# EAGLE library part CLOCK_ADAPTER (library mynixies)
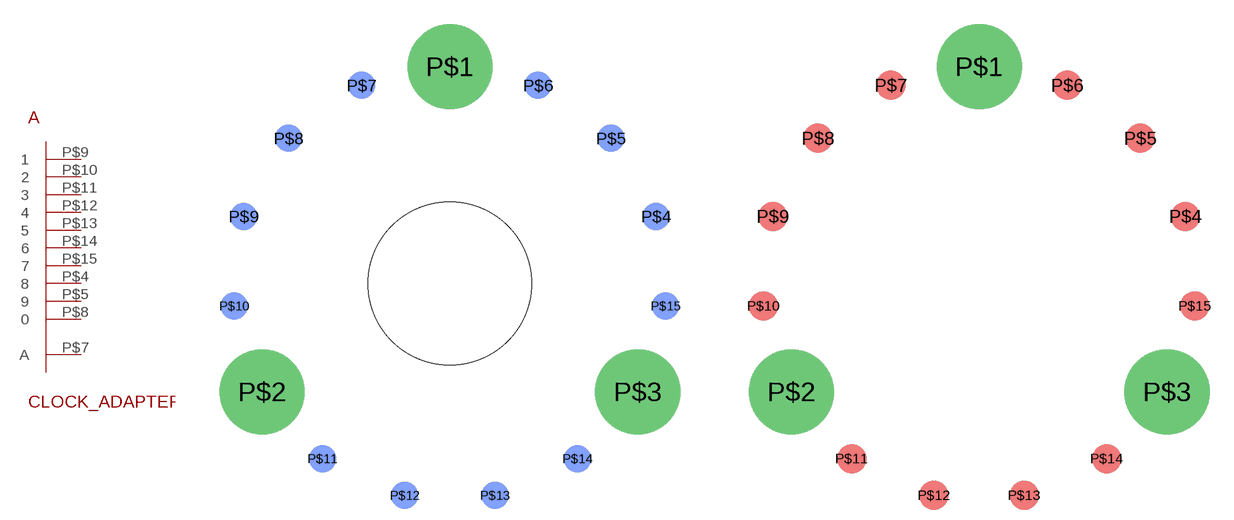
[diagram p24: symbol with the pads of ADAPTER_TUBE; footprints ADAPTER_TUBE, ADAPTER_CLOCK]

Designator prefix A

## CLOCK_ADAPTERTUBE  [ADAPTER_TUBE]
P$4  8  pas
P$5  9  pas
P$7  A  pas
P$8  0  pas
P$9  1  pas
P$10  2  pas
P$11  3  pas
P$12  4  pas
P$13  5  pas
P$14  6  pas
P$15  7  pas

## CLOCK_ADAPTERCLOCK  [ADAPTER_CLOCK]
Pads as for ADAPTER_TUBE

## Footprint ADAPTER_TUBE (pad centres in mm)
drill 2.2 pad 5.3: P$1 0,13.5; P$2 -11.691,-6.75; P$3 11.691,-6.75
smd 1.7 x 1.7 bottom: P$4 12.839,4.172; P$5 10.032,9.033; P$6 5.491,12.333; P$7 -5.491,12.333; P$8 -10.032,9.033; P$9 -12.839,4.172; P$10 -13.426,-1.411; P$11 -7.935,-10.922; P$12 -2.807,-13.205; P$13 2.807,-13.205; P$14 7.935,-10.922; P$15 13.426,-1.411
hole 10.16 at 0,0

## Footprint ADAPTER_CLOCK (pad centres in mm)
drill 3 pad 5.3: P$1 0,13.5; P$2 -11.691,-6.75; P$3 11.691,-6.75
smd 1.829 x 1.829: P$4 12.839,4.172; P$5 10.032,9.033; P$6 5.491,12.333; P$7 -5.491,12.333; P$8 -10.032,9.033; P$9 -12.839,4.172; P$10 -13.426,-1.411; P$11 -7.935,-10.922; P$12 -2.807,-13.205; P$13 2.807,-13.205; P$14 7.935,-10.922; P$15 13.426,-1.411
